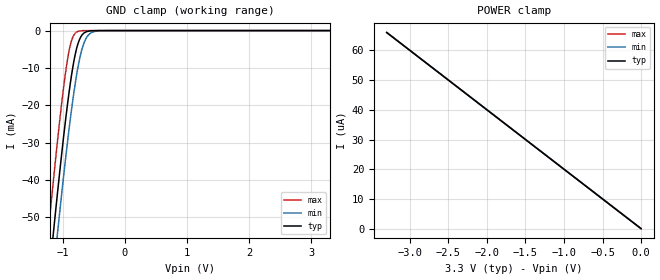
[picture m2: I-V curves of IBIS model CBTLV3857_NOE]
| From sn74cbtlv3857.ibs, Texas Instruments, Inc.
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[Model]   CBTLV3857_NOE
Model_type  Input
Vinl = 1.0
Vinh = 1.33
| variable   typ   min   max
C_comp   1.52pF   1.33pF   1.94pF
[Temperature Range]   40   100   -40
| Ambient temperature   25   85   -40
[Voltage range]   3.3   3   3.6
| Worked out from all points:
|   GND clamp passes 1 mA (typ) near -0.68 V on its own axis
[GND Clamp]
| CBTLV3857A_NOE
|   Voltage   I(typ)   I(min)   I(max)
-3.3V     -452.3mA   -461.2mA   -441.6mA
-1.235V   -68.47mA   -79.32mA   -54.53mA
-1.155V   -55.02mA   -65.9mA    -41.02mA
-1.085V   -43.65mA   -54.48mA   -29.72mA
-990mV    -29.08mA   -39.65mA   -15.78mA
-910mV    -18.08mA   -28.05mA   -6.523mA
-845mV    -10.58mA   -19.54mA   -2.069mA
-770mV    -4.399mA   -11.26mA   -340.3uA
-705mV    -1.577mA   -5.93mA    -59.98uA
-645mV    -520uA     -2.804mA   -11.73uA
-480mV    -19.14uA   -210.8uA   -129.8nA
3.3V      1.114nA    59.61nA    6.193pA
[POWER Clamp]
| CBTLV3857_NOE
|   Voltage   I(typ)   I(min)   I(max)
-3.3V     66uA       66.06uA    66uA
-3.295V   65.9uA     65.96uA    65.9uA
-1.25V    25uA       25.06uA    25uA
-48.03fV  1.153nA    59.68nA    36.96pA
